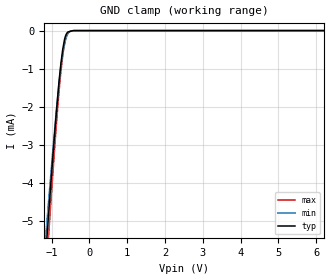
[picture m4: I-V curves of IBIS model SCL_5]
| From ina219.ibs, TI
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|   5V SCL Input Model
[Model] SCL_5
Model_type Input
| Signals  SCL
Vinl = 1.5
Vinh = 3.5
|   typ   min   max
C_comp   1.1266090e-12   1.2181950e-12   1.0025750e-12
[Voltage Range]   5   4.5   5.5
[Temperature Range]   27   85   -25
[Power Clamp Reference]   5   4.5   5.5
[GND Clamp Reference]   0   0   0
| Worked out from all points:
|   GND clamp passes 1 mA (typ) near -0.77 V on its own axis
[GND Clamp]
|   Voltage   I(typ)   I(min)   I(max)
-5V       -62.83mA   -55.74mA   -71.99mA
-1.149V   -5.796mA   -5.326mA   -6.432mA
-1.103V   -5.151mA   -4.758mA   -5.744mA
-1.087V   -4.935mA   -4.565mA   -5.508mA
-1.03V    -4.17mA    -3.891mA   -4.664mA
-893.3mV  -2.381mA   -2.31mA    -2.737mA
-764.8mV  -966.2uA   -1.042mA   -1.195mA
-673.2mV  -317.8uA   -428.5uA   -442.4uA
-624.3mV  -123.5uA   -220.7uA   -202.8uA
-570.1mV  -36.84uA   -85.98uA   -76.98uA
-404.8mV  -844.2nA   -802nA     -777.5nA
9.985V    0A         0A         0A
[POWER Clamp]
|   SCR cell for ESD function. Effects occurr above VDD x 2
|   Voltage   I(typ)   I(min)   I(max)
-5V       0A         0A         0A
0V        0A         0A         0A
10V       0A         0A         0A
